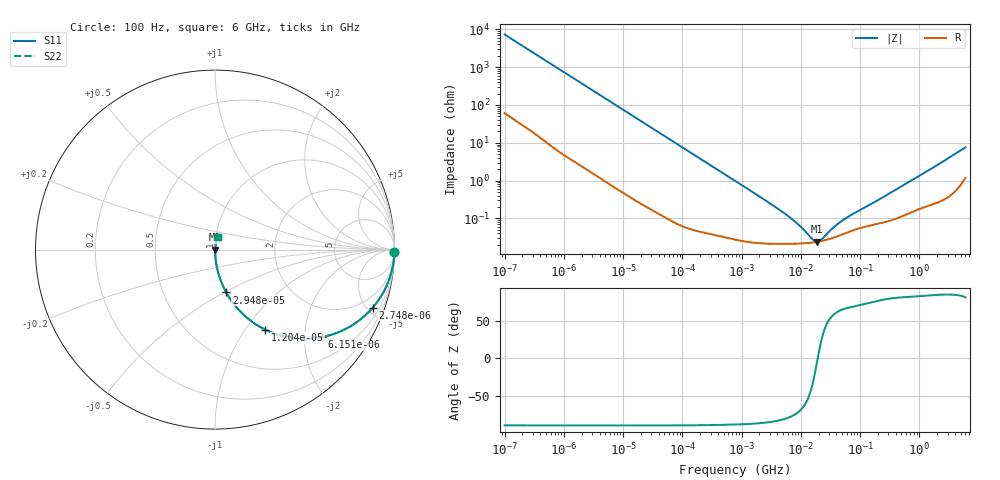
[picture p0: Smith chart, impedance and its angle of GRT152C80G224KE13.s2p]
!Murata Part Number: GRT152C80G224KE13
!These Parameters are Measured in Series Mode Connection
!Data Generated on Jun 19, 2026
!  o--ll--o
!Port1  Port2
!  o------o
!Operation Temp=25[degC], DC Bias Voltage=0[V]
!Freq. Start=100[Hz] Stop=6[GHz] 401[Steps]
# Hz S RI R 50
!Freq.(Hz) S11(Real) S11(Imag) S21(Real) S21(Imag) S12(Real) S12(Imag) S22(Real) S22(Imag)
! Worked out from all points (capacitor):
!   401 points, 100 Hz to 6 GHz, reference 50 ohm
!   read as one part in series: C = 216 nF near 109 Hz
!   lowest |Z| = 24 mohm at 18.61 MHz (marker M1)
!   series resonance near 19.3 MHz, so ESL is about 310 pH
!   S11 on the Smith chart (normalised r, x): 100 Hz: open; 2.748 kHz: 1.03, -5.43; 6.151 kHz: 1.02, -2.43; 12.04 kHz: 1.01, -1.25; 29.48 kHz: 1.00, -0.51; 6 GHz: 1.02, +0.15
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100  0.9997 -0.0136  0.000297 0.0136  0.000297 0.0136  0.9997 -0.0136
600  0.993 -0.0802  0.00702 0.0802  0.00702 0.0802  0.993 -0.0802
2008  0.9309 -0.2504  0.0691 0.2504  0.0691 0.2504  0.9309 -0.2504
2748  0.879 -0.3229  0.121 0.3229  0.121 0.3229  0.879 -0.3229
4111  0.7663 -0.4201  0.2337 0.4201  0.2337 0.4201  0.7663 -0.4201
6151  0.5963 -0.4875  0.4037 0.4875  0.4037 0.4875  0.5963 -0.4875
8416  0.4426 -0.4936  0.5574 0.4936  0.5574 0.4936  0.4426 -0.4936
12041  0.281 -0.4464  0.719 0.4464  0.719 0.4464  0.281 -0.4464
18841  0.1389 -0.3427  0.8611 0.3427  0.8611 0.3427  0.1389 -0.3427
29482  0.0626 -0.239  0.9374 0.239  0.9374 0.239  0.0626 -0.239
40335  0.0349 -0.1802  0.9651 0.1802  0.9651 0.1802  0.0349 -0.1802
129199  0.00394 -0.0583  0.9961 0.0583  0.9961 0.0583  0.00394 -0.0583
774597  0.00037 -0.00984  0.9996 0.00984  0.9996 0.00984  0.00037 -0.00984
6075234  0.000212 -0.00113  0.9998 0.00113  0.9998 0.00113  0.000212 -0.00113
9506416  0.000215 -0.000607  0.9998 0.000607  0.9998 0.000607  0.000215 -0.000607
1.555665e7  0.000229 -0.00017  0.9998 0.00017  0.9998 0.00017  0.000229 -0.00017
1.86079e7  0.000238 -2.82e-05  0.9998 2.82e-05  0.9998 2.82e-05  0.000238 -2.82e-05
2.225763e7  0.000251 0.000111  0.9997 -0.000111  0.9997 -0.000111  0.000251 0.000111
3.64232e7  0.000311 0.000504  0.9997 -0.000504  0.9997 -0.000504  0.000311 0.000504
5.449875e7  0.000394 0.000867  0.9996 -0.000867  0.9996 -0.000867  0.000394 0.000867
3.124326e8  0.000872 0.00445  0.9991 -0.00445  0.9991 -0.00445  0.000872 0.00445
6e9  0.0169 0.0725  0.9831 -0.0725  0.9831 -0.0725  0.0169 0.0725
